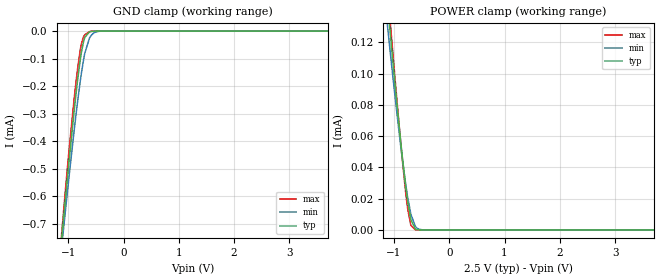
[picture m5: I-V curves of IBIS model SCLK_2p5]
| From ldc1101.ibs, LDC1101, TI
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|   Model
[Model]   SCLK_2p5
Model_type   Input
Vinl = 0.75
Vinh = 1.75
|   typ   min   max
C_comp   0.346pF   0.312pF   0.398pF
[Voltage Range]   2.5   2.25   2.75
[Temperature Range]   27   125   -40
[Power Clamp Reference]   2.5   2.25   2.75
[GND Clamp Reference]   0   0   0
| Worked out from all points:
|   GND clamp passes 1 mA (typ) near -1.23 V on its own axis
[GND Clamp]
|   Voltage   I(typ)   I(min)   I(max)
-2.5V     -3.863mA   -3.619mA   -4.127mA
-1.195V   -916.4uA   -931.6uA   -910.4uA
-1.052V   -611.3uA   -654.4uA   -579.8uA
-895mV    -293.8uA   -364.2uA   -249.2uA
-827.5mV  -173.1uA   -250.5uA   -131.8uA
-782.5mV  -104uA     -181.5uA   -68.3uA
-760mV    -74.93uA   -150.1uA   -44.62uA
-700mV    -23uA      -80.18uA   -13.11uA
-617.5mV  -3.077uA   -26.24uA   -2.21uA
-527.5mV  -287.2nA   -5.752uA   -130.3nA
-377.5mV  0A         -191.3nA   0A
5V        0A         0A         0A
[POWER Clamp]
|   Voltage   I(typ)   I(min)   I(max)
-2.5V     708.3uA    627.2uA    773.8uA
-1.248V   195.4uA    174.3uA    209.6uA
-1.067V   125.3uA    113.1uA    132.3uA
-1.06V    122.5uA    110.6uA    129.1uA
-1.052V   119.6uA    108.1uA    125.9uA
-872.5mV  54.14uA    51.68uA    53.05uA
-767.5mV  21.82uA    24.01uA    17.35uA
-700mV    7.467uA    10.89uA    3.67uA
-617.5mV  871.8nA    2.528uA    163.4nA
-542.5mV  78.89nA    465.3nA    3.614nA
-407.5mV  0A         11.88nA    0A
5V        0A         0A         0A
